FUNCTION "COM_FEEDER" : VOID
TITLE =FEEDER MANAGEMENT
VERSION : 0.1

BEGIN
NETWORK
TITLE =FEEDER ON
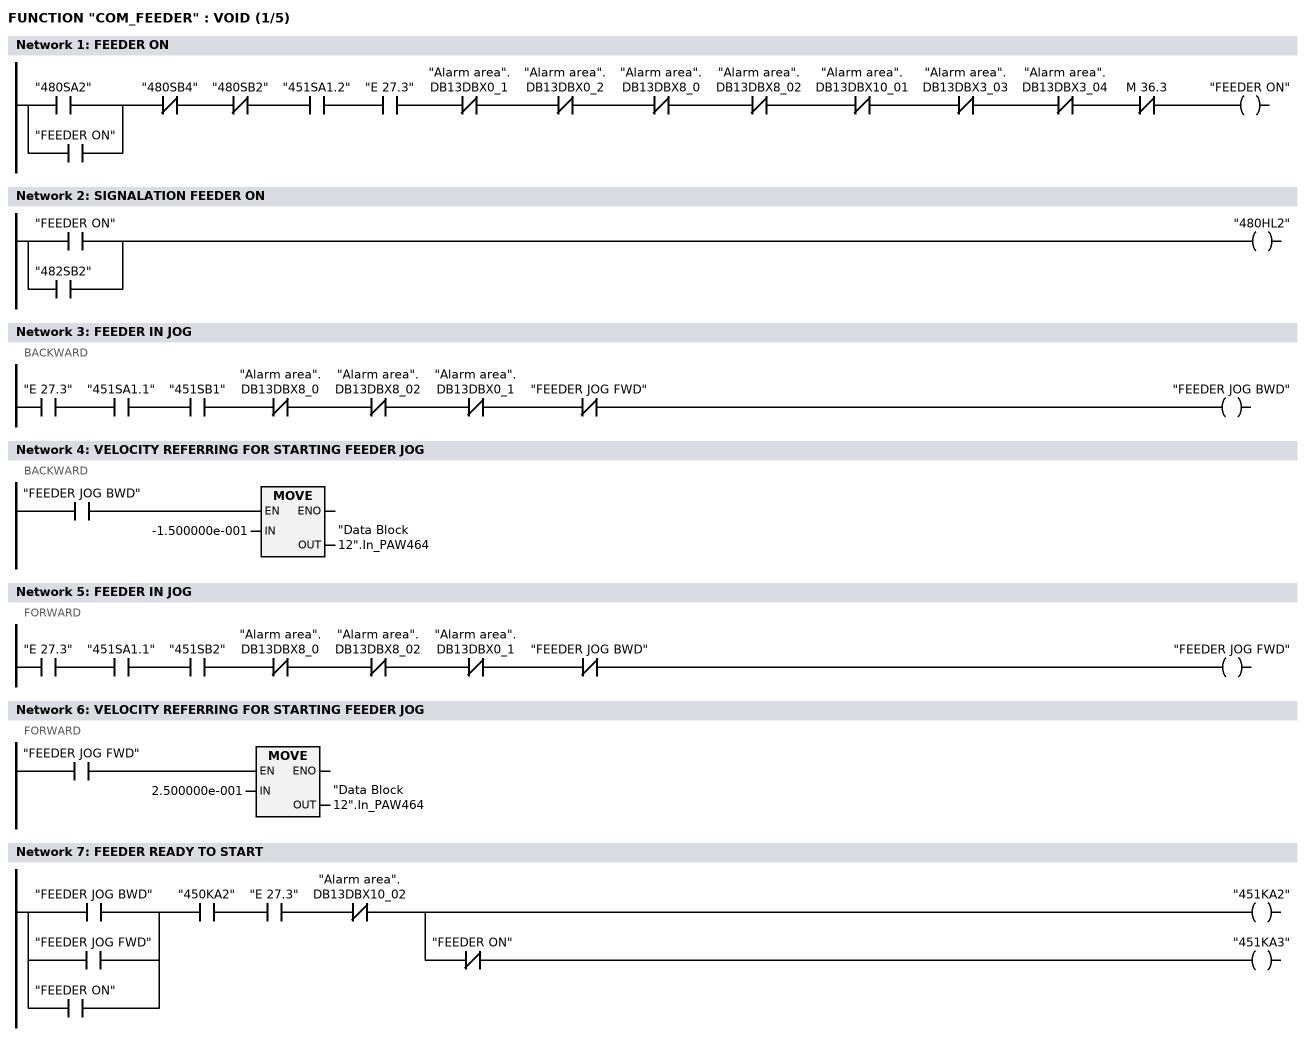
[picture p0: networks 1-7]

      U(    ;
      O     "480SA2";
      O     "FEEDER ON";
      )     ;
      UN    "480SB4";
      UN    "480SB2";
      U     "451SA1.2";
      U     "E      27.3";
      UN    "Alarm area".DB13DBX0_1;
      UN    "Alarm area".DB13DBX0_2;
      UN    "Alarm area".DB13DBX8_0;
      UN    "Alarm area".DB13DBX8_02;
      UN    "Alarm area".DB13DBX10_01;
      UN    "Alarm area".DB13DBX3_03;
      UN    "Alarm area".DB13DBX3_04;
      UN    M     36.3;
      =     "FEEDER ON";
NETWORK
TITLE =SIGNALATION FEEDER ON


      O     "FEEDER ON";
      O     "482SB2";
      =     "480HL2";
NETWORK
TITLE =FEEDER IN JOG
//BACKWARD
      U     "E      27.3";
      U     "451SA1.1";
      U     "451SB1";
      UN    "Alarm area".DB13DBX8_0;
      UN    "Alarm area".DB13DBX8_02;
      UN    "Alarm area".DB13DBX0_1;
      UN    "FEEDER JOG FWD";
      =     "FEEDER JOG BWD";

NETWORK
TITLE =VELOCITY REFERRING FOR STARTING FEEDER JOG
//BACKWARD
      U     "FEEDER JOG BWD";
      SPBN  JOGB;
      L     -1.500000e-001;
      T     "Data Block 12".In_PAW464;
JOGB: NOP   0;

NETWORK
TITLE =FEEDER IN JOG
//FORWARD
      U     "E      27.3";
      U     "451SA1.1";
      U     "451SB2";
      UN    "Alarm area".DB13DBX8_0;
      UN    "Alarm area".DB13DBX8_02;
      UN    "Alarm area".DB13DBX0_1;
      UN    "FEEDER JOG BWD";
      =     "FEEDER JOG FWD";

NETWORK
TITLE =VELOCITY REFERRING FOR STARTING FEEDER JOG
//FORWARD
      U     "FEEDER JOG FWD";
      SPBN  JOGF;
      L     2.500000e-001;
      T     "Data Block 12".In_PAW464;
JOGF: NOP   0;

NETWORK
TITLE =FEEDER READY TO START

      U(    ;
      O     "FEEDER JOG BWD";
      O     "FEEDER JOG FWD";
      O     "FEEDER ON";
      )     ;
      U     "450KA2";
      U     "E      27.3";
      UN    "Alarm area".DB13DBX10_02;
      =     L      0.0;
      U     L      0.0;
      BLD   102;
      =     "451KA2";
      U     L      0.0;
      UN    "FEEDER ON";
      =     "451KA3";
NETWORK
TITLE =START POSITIONING FEEDER
//SINGLE STROKE / CONTINUOUS
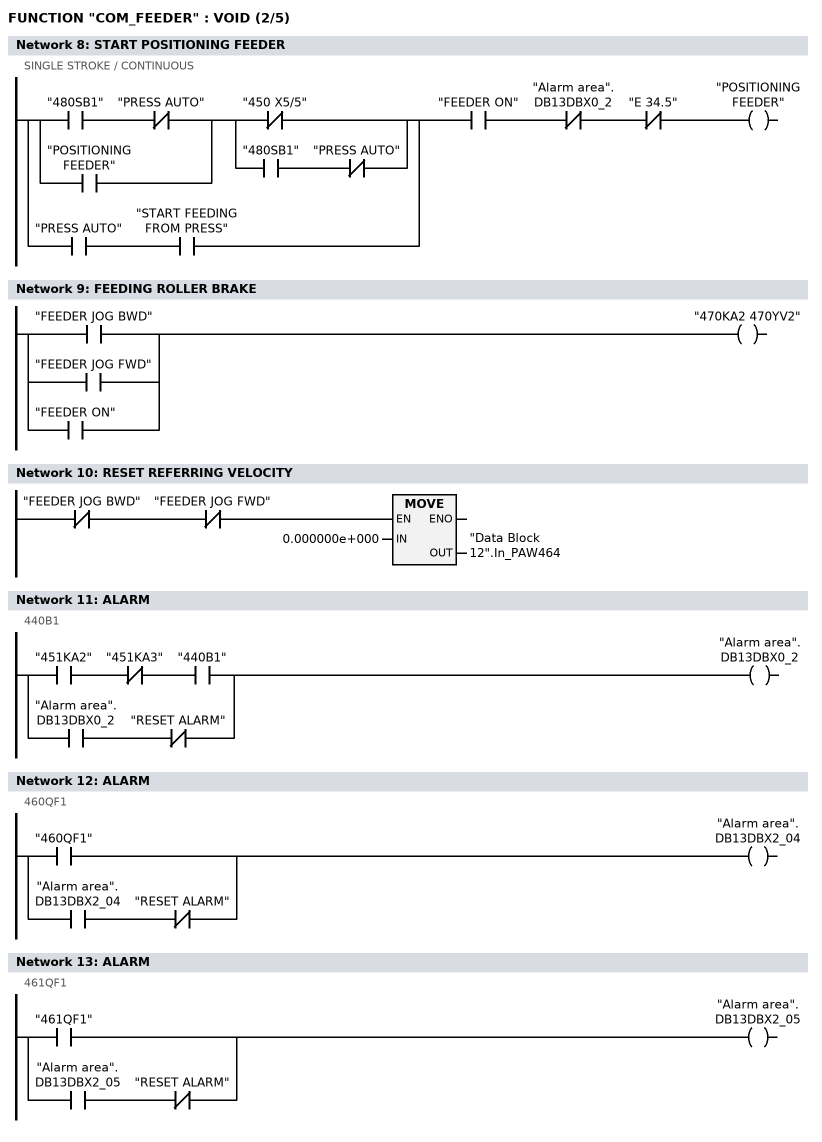
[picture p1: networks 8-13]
      U(    ;
      U(    ;
      U     "480SB1";
      UN    "PRESS AUTO";
      O     "POSITIONING FEEDER";
      )     ;
      U(    ;
      ON    "450 X5/5";
      O     ;
      U     "480SB1";
      UN    "PRESS AUTO";
      )     ;
      O     ;
      U     "PRESS AUTO";
      U     "START FEEDING FROM PRESS";
      )     ;
      U     "FEEDER ON";
      UN    "Alarm area".DB13DBX0_2;
      UN    "E      34.5";
      =     "POSITIONING FEEDER";
NETWORK
TITLE =FEEDING ROLLER BRAKE

      O     "FEEDER JOG BWD";
      O     "FEEDER JOG FWD";
      O     "FEEDER ON";
      =     "470KA2 470YV2";
NETWORK
TITLE =RESET REFERRING VELOCITY

      UN    "FEEDER JOG BWD";
      UN    "FEEDER JOG FWD";
      SPBN  RES0;
      L     0.000000e+000;
      T     "Data Block 12".In_PAW464;
RES0: NOP   0;


NETWORK
TITLE =ALARM
//440B1
      U     "451KA2";
      UN    "451KA3";
      U     "440B1";
      O     ;
      U     "Alarm area".DB13DBX0_2;
      UN    "RESET ALARM";
      =     "Alarm area".DB13DBX0_2;
NETWORK
TITLE =ALARM
//460QF1
      O     "460QF1";
      O     ;
      U     "Alarm area".DB13DBX2_04;
      UN    "RESET ALARM";
      =     "Alarm area".DB13DBX2_04;


NETWORK
TITLE =ALARM
//461QF1
      O     "461QF1";
      O     ;
      U     "Alarm area".DB13DBX2_05;
      UN    "RESET ALARM";
      =     "Alarm area".DB13DBX2_05;

NETWORK
TITLE =ALARM
//FEEDER MASTER READY
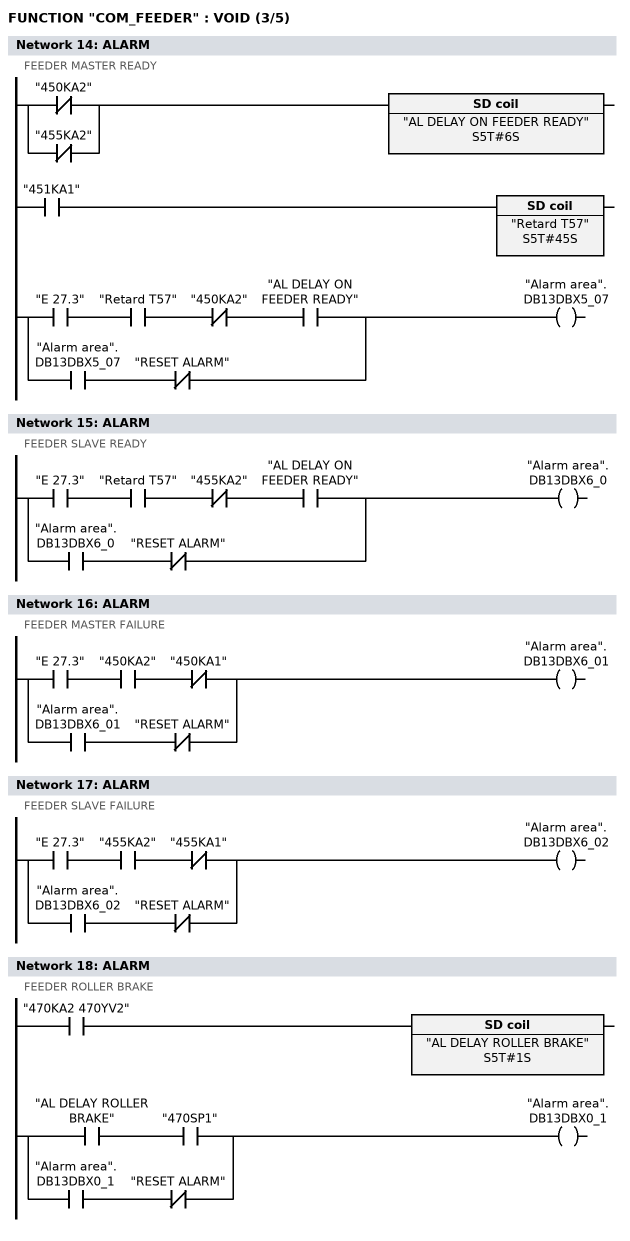
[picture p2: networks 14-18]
      ON    "450KA2";
      ON    "455KA2";
      L     S5T#6S;
      SE    "AL DELAY ON FEEDER READY";

      U     "451KA1";
      L     S5T#45S;
      SE    "Retard T57";

      U     "E      27.3";
      U     "Retard T57";
      UN    "450KA2";
      U     "AL DELAY ON FEEDER READY";
      O     ;
      U     "Alarm area".DB13DBX5_07;
      UN    "RESET ALARM";
      =     "Alarm area".DB13DBX5_07;

NETWORK
TITLE =ALARM
//FEEDER SLAVE READY
      U     "E      27.3";
      U     "Retard T57";
      UN    "455KA2";
      U     "AL DELAY ON FEEDER READY";
      O     ;
      U     "Alarm area".DB13DBX6_0;
      UN    "RESET ALARM";
      =     "Alarm area".DB13DBX6_0;

NETWORK
TITLE =ALARM
//FEEDER MASTER FAILURE
      U     "E      27.3";
      U     "450KA2";
      UN    "450KA1";
      O     ;
      U     "Alarm area".DB13DBX6_01;
      UN    "RESET ALARM";
      =     "Alarm area".DB13DBX6_01;

NETWORK
TITLE =ALARM
//FEEDER SLAVE FAILURE
      U     "E      27.3";
      U     "455KA2";
      UN    "455KA1";
      O     ;
      U     "Alarm area".DB13DBX6_02;
      UN    "RESET ALARM";
      =     "Alarm area".DB13DBX6_02;

NETWORK
TITLE =ALARM
//FEEDER ROLLER BRAKE
      U     "470KA2 470YV2";
      L     S5T#1S;
      SE    "AL DELAY ROLLER BRAKE";

      U     "AL DELAY ROLLER BRAKE";
      U     "470SP1";
      O     ;
      U     "Alarm area".DB13DBX0_1;
      UN    "RESET ALARM";
      =     "Alarm area".DB13DBX0_1;

NETWORK
TITLE =ALARM
//450KM1
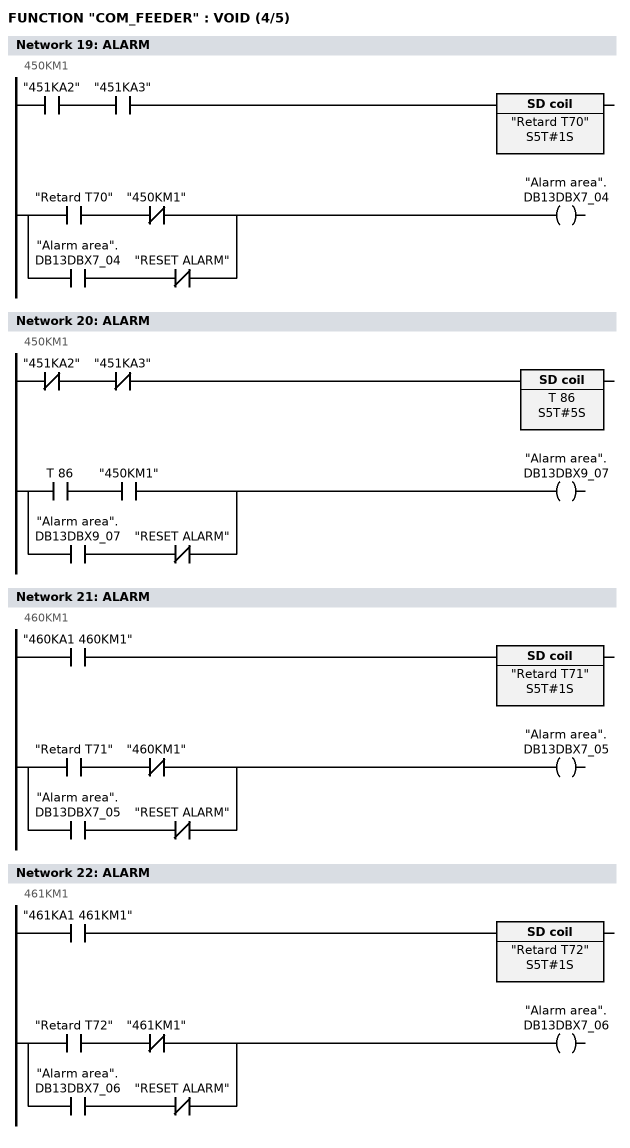
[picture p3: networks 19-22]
      U     "451KA2";
      U     "451KA3";
      L     S5T#1S;
      SE    "Retard T70";

      U     "Retard T70";
      UN    "450KM1";
      O     ;
      U     "Alarm area".DB13DBX7_04;
      UN    "RESET ALARM";
      =     "Alarm area".DB13DBX7_04;

NETWORK
TITLE =ALARM
//450KM1
      UN    "451KA2";
      UN    "451KA3";
      L     S5T#5S;
      SE    T     86;

      U     T     86;
      U     "450KM1";
      O     ;
      U     "Alarm area".DB13DBX9_07;
      UN    "RESET ALARM";
      =     "Alarm area".DB13DBX9_07;

NETWORK
TITLE =ALARM
//460KM1
      U     "460KA1 460KM1";

      L     S5T#1S;
      SE    "Retard T71";

      U     "Retard T71";
      UN    "460KM1";
      O     ;
      U     "Alarm area".DB13DBX7_05;
      UN    "RESET ALARM";
      =     "Alarm area".DB13DBX7_05;

NETWORK
TITLE =ALARM
//461KM1
      U     "461KA1 461KM1";

      L     S5T#1S;
      SE    "Retard T72";

      U     "Retard T72";
      UN    "461KM1";
      O     ;
      U     "Alarm area".DB13DBX7_06;
      UN    "RESET ALARM";
      =     "Alarm area".DB13DBX7_06;

NETWORK
TITLE =CUMULATIVE ALARM FEEDER
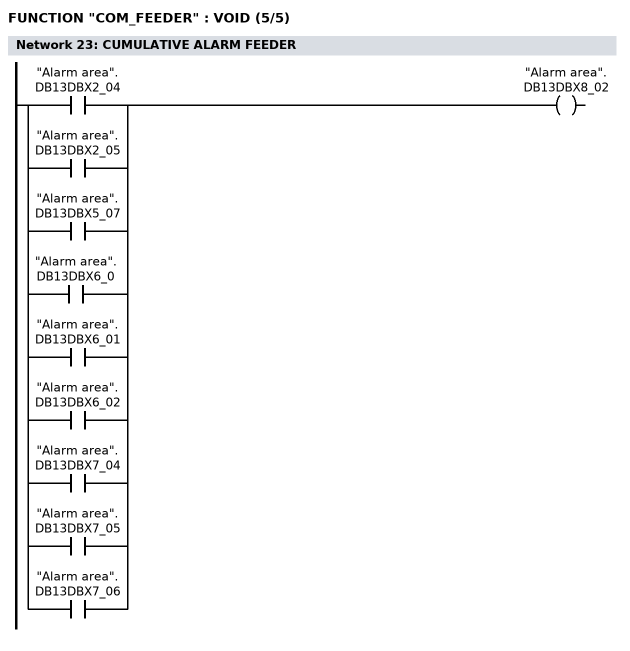
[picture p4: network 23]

      O     "Alarm area".DB13DBX2_04;
      O     "Alarm area".DB13DBX2_05;
      O     "Alarm area".DB13DBX5_07;
      O     "Alarm area".DB13DBX6_0;
      O     "Alarm area".DB13DBX6_01;
      O     "Alarm area".DB13DBX6_02;
      O     "Alarm area".DB13DBX7_04;
      O     "Alarm area".DB13DBX7_05;
      O     "Alarm area".DB13DBX7_06;
      =     "Alarm area".DB13DBX8_02;

END_FUNCTION

